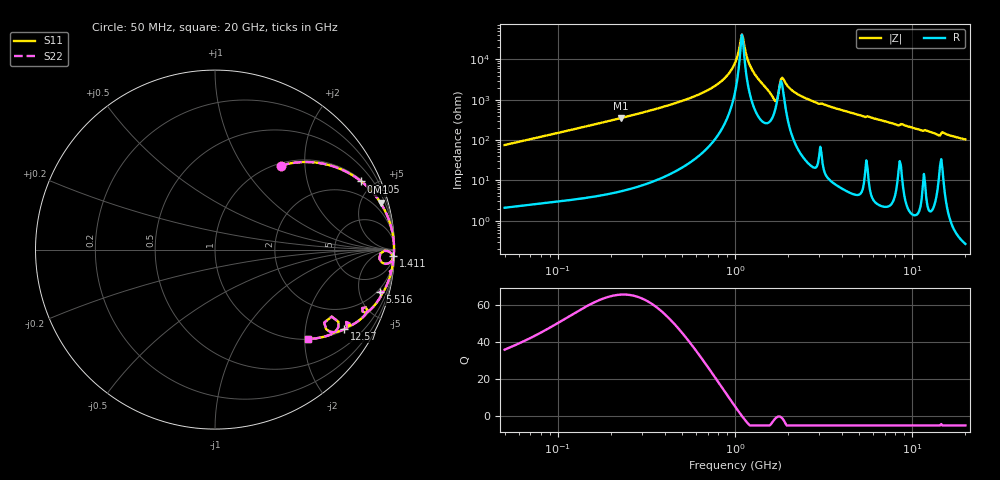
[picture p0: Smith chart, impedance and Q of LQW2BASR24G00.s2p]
!Murata Part Number: LQW2BASR24G00
!These Parameters are Measured in Series Mode Connection
!  o--[Z]--o
!Port1  Port2
!  o-------o
!Freq. Start=50[MHz] Stop=20[GHz], 401[Steps]
# Hz S RI R 50
!Freq.(Hz) S11(Real) S11(Imag) S21(Real) S21(Imag) S12(Real) S12(Imag) S22(Real) S22(Imag)
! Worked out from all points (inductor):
!   401 points, 50 MHz to 20 GHz, reference 50 ohm
!   read as one part in series: L = 239 nH near 51.52 MHz
!   highest Q = 65.9 at 227 MHz (marker M1), where L = 247 nH
!   self-resonance near 1.094 GHz
!   S11 on the Smith chart (normalised r, x): 50 MHz: 1.04, +1.51; 140.5 MHz: 1.07, +4.26; 1.411 GHz: 7, -52; 5.516 GHz: 1.63, -7.53; 12.57 GHz: 1.03, -3.22; 20 GHz: 1.01, -2.08
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5e7  0.3661 0.4681  0.6339 -0.4681  0.6339 -0.4681  0.3661 0.4681
1.364002e8  0.8059 0.387  0.1941 -0.387  0.1941 -0.387  0.8059 0.387
1.405482e8  0.8152 0.3798  0.1848 -0.3798  0.1848 -0.3798  0.8152 0.3798
2.269813e8  0.9221 0.2606  0.0779 -0.2606  0.0779 -0.2606  0.9221 0.2606
3.721004e8  0.9723 0.1558  0.0277 -0.1558  0.0277 -0.1558  0.9723 0.1558
7.411344e8  0.9953 0.0501  0.00467 -0.0501  0.00467 -0.0501  0.9953 0.0501
8.870719e8  0.9971 0.0271  0.0029 -0.0271  0.0029 -0.0271  0.9971 0.0271
1e9  0.9976 0.0119  0.00238 -0.0119  0.00238 -0.0119  0.9976 0.0119
1.077769e9  0.9977 0.00226  0.00235 -0.00226  0.00235 -0.00226  0.9977 0.00226
1.110545e9  0.9976 -0.00166  0.0024 0.00166  0.0024 0.00166  0.9976 -0.00166
1.214974e9  0.9971 -0.0138  0.00288 0.0138  0.00288 0.0138  0.9971 -0.0138
1.411297e9  0.9943 -0.0373  0.00573 0.0373  0.00573 0.0373  0.9943 -0.0373
1.664083e9  0.9502 -0.0796  0.0498 0.0796  0.0498 0.0796  0.9502 -0.0796
1.714689e9  0.9154 -0.0503  0.0846 0.0503  0.0846 0.0503  0.9154 -0.0503
1.820564e9  0.9738 -0.0135  0.0262 0.0135  0.0262 0.0135  0.9738 -0.0135
1.875929e9  0.9853 -0.0265  0.0147 0.0265  0.0147 0.0265  0.9853 -0.0265
2.146657e9  0.9922 -0.0622  0.0078 0.0622  0.0078 0.0622  0.9922 -0.0622
2.728004e9  0.9863 -0.105  0.0137 0.105  0.0137 0.105  0.9863 -0.105
5.515528e9  0.9173 -0.2368  0.0827 0.2368  0.0827 0.2368  0.9173 -0.2368
7.442007e9  0.8796 -0.3212  0.1204 0.3212  0.1204 0.3212  0.8796 -0.3212
1.257102e10  0.7198 -0.4438  0.2802 0.4438  0.2802 0.4438  0.7198 -0.4438
2e10  0.5184 -0.4984  0.4816 0.4984  0.4816 0.4984  0.5184 -0.4984
